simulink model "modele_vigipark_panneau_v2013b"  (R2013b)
settings: Solver=ode15s  StartTime=0.0  StopTime=3600  RelTol=1e-3
undefined symbols (not defined in the file): IRR
libraries: nesl_utility x4, fl_lib x3, elec_lib x2

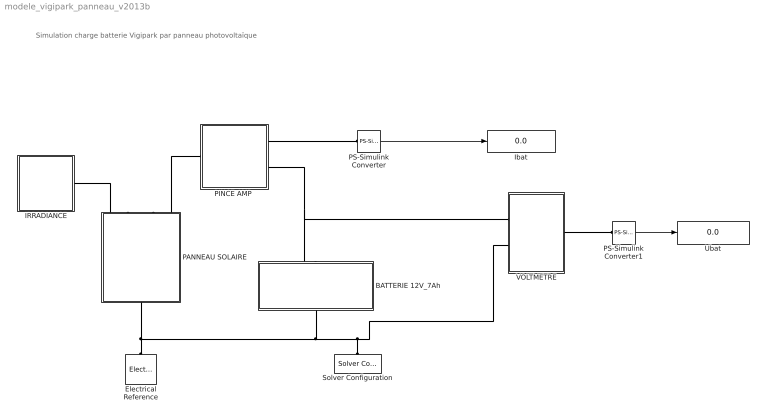
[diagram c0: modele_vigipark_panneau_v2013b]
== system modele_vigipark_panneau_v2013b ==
  note: Simulation charge batterie Vigipark par panneau photovoltaïque
  BATTERIE 12V_7Ah : Subsystem
  Electrical Reference : fl_lib/Electrical/Electrical Elements/Electrical Reference  i_Log=off  LocalVarNames=|i  LocalVarDescs=|i  LocalVarLogging=0
  IRRADIANCE : Subsystem
  Ibat : Display
  PANNEAU SOLAIRE : Subsystem
  "PINCE AMP " : Subsystem
  PS-Simulink Converter : nesl_utility/PS-Simulink Converter  PhysicalDomain=network_engine_domain  SubClassName=ps_output  LeftPortType=input  RightPortType=output  PseudoPeriodic=off  Frequencies=[]  Unit=A  AffineConversion=off
  PS-Simulink Converter1 : nesl_utility/PS-Simulink Converter  PhysicalDomain=network_engine_domain  SubClassName=ps_output  LeftPortType=input  RightPortType=output  PseudoPeriodic=off  Frequencies=[]  Unit=V  AffineConversion=off
  Solver Configuration : nesl_utility/Solver Configuration  PhysicalDomain=network_engine_domain  SubClassName=solver  LeftPortType=input  RightPortType=generic  Accelerate=off  Tones=[]  Harmonics=[]  SimulateNoise=off  Profile=off  UseLocalSampling=off  EnableSwitchedLinearOptims=on  FrequencyDomain=off  UseCCode=off  RelTol=0.001  AbsTol=1e-06  MinStep=1e-09  ToWorkspace=off  DoDC=off  ResidualTolerance=1e-9  UseLocalSolver=off  LocalSolverChoice=NE_BACKWARD_EULER_ADVANCER  LocalSolverSampleTime=.001  DoFixedCost=off  MaxNonlinIter=3  MaxModeIter=2  LinearAlgebra=Sparse  DelaysMemoryBudget=1024
  Ubat : Display
  VOLTMETRE : Subsystem
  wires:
  PS-Simulink Converter/1 -> Ibat/1
  PS-Simulink Converter1/1 -> Ubat/1
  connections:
  "PINCE AMP "/RConn2 -- BATTERIE 12V_7Ah/LConn1 -- VOLTMETRE/RConn1
  Solver Configuration/RConn1 -- PANNEAU SOLAIRE/LConn1 -- Electrical Reference/LConn1 -- BATTERIE 12V_7Ah/RConn1 -- VOLTMETRE/RConn2
  IRRADIANCE/LConn1 -- PANNEAU SOLAIRE/RConn1
  "PINCE AMP "/RConn1 -- PS-Simulink Converter/LConn1
  "PINCE AMP "/LConn1 -- PANNEAU SOLAIRE/RConn2
  VOLTMETRE/LConn1 -- PS-Simulink Converter1/LConn1

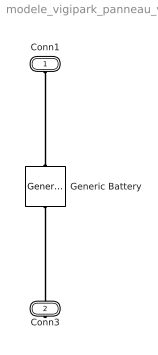
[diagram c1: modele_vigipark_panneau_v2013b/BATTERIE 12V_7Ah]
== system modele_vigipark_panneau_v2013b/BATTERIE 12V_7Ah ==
  Generic Battery : elec_lib/Sources/Generic Battery  Vnom=12 V  R1=0.018 Ohm  prm_AH=2  AH=7 hr*A  AH0=7 hr*A  V1=11.5 V  AH1=3.5 hr*A  prm_R2=1  R2=2e+3 Ohm  LocalVarLogging=[]
  Conn1 : PMIOPort  Port=1  Side=Left
  Conn3 : PMIOPort  Port=2  Side=Right
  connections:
  Conn1/RConn1 -- Generic Battery/LConn1
  Conn3/RConn1 -- Generic Battery/RConn1

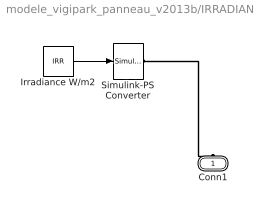
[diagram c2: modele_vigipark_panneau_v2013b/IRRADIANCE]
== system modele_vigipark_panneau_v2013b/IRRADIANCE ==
  Irradiance W/m2 : Constant  Value=IRR
  Simulink-PS Converter : nesl_utility/Simulink-PS Converter  PhysicalDomain=network_engine_domain  SubClassName=ps_input  LeftPortType=input  RightPortType=output  PseudoPeriodic=off  Frequencies=[]  NoiseDistribution=none  NoiseParameters=[]  Unit=1  AffineConversion=off  InputFiltering=off  SimscapeFilterOrder=1  InputFilterTimeConstant=.001  UdotUserProvided=1
  Conn1 : PMIOPort  Port=1  Side=Left
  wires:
  Irradiance W/m2/1 -> Simulink-PS Converter/1
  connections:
  Simulink-PS Converter/RConn1 -- Conn1/RConn1

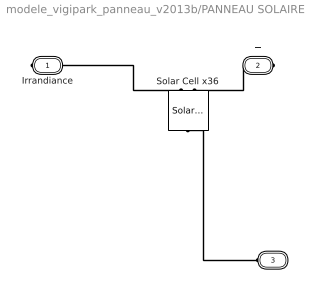
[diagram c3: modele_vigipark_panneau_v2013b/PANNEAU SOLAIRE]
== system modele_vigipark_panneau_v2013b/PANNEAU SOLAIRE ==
  Solar Cell x36 : elec_lib/Sources/Solar Cell  prm=1  Isc=0.7 A  Voc=0.569444 V  Is=1e-6 A  Is2=0 A  Iph=7.34 A  Ir0=1000 W/m^2  ec=1.5  N2=2  Rs=0 Ohm  Rp=Inf Ohm  N_series=36  TIPH1=0 1/K  EG=1.11 eV  TXIS1=3  TXIS2=3  TRS1=0  TRP1=0  Tmeas=25 C  TFIXED=temp C  LocalVarLogging=[]  thermal_mass=100 J/K  initial_temperature=25 C
  Irrandiance : PMIOPort  Tag=PMCPort  Port=1  Side=Right
  + : PMIOPort  Tag=PMCPort  Port=2  Side=Right
  - : PMIOPort  Tag=PMCPort  Port=3  Side=Left
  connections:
  Irrandiance/RConn1 -- Solar Cell x36/LConn1
  +/RConn1 -- Solar Cell x36/LConn2
  -/RConn1 -- Solar Cell x36/RConn1

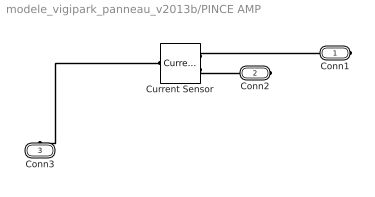
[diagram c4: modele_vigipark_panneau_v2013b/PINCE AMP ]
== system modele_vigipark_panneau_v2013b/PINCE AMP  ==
  Current Sensor : fl_lib/Electrical/Electrical Sensors/Current Sensor  i1_Log=off  v1_Log=off  LocalVarNames=|i1|v1  LocalVarDescs=|i1|v1  LocalVarLogging=[0 0]
  Conn1 : PMIOPort  Port=1  Side=Right
  Conn2 : PMIOPort  Port=2  Side=Right
  Conn3 : PMIOPort  Port=3  Side=Left
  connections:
  Current Sensor/LConn1 -- Conn3/RConn1
  Current Sensor/RConn1 -- Conn1/RConn1
  Current Sensor/RConn2 -- Conn2/RConn1

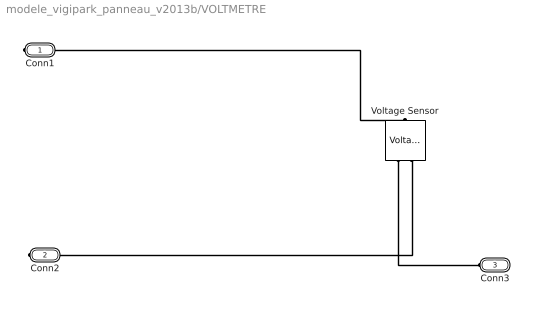
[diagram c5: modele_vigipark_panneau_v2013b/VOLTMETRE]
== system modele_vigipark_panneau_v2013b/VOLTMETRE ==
  Voltage Sensor : fl_lib/Electrical/Electrical Sensors/Voltage Sensor  i1_Log=off  v1_Log=off  LocalVarNames=|i1|v1  LocalVarDescs=|i1|v1  LocalVarLogging=[0 0]
  Conn1 : PMIOPort  Port=1  Side=Right
  Conn2 : PMIOPort  Port=2  Side=Right
  Conn3 : PMIOPort  Port=3  Side=Left
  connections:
  Voltage Sensor/RConn1 -- Conn3/RConn1
  Conn1/RConn1 -- Voltage Sensor/LConn1
  Voltage Sensor/RConn2 -- Conn2/RConn1
